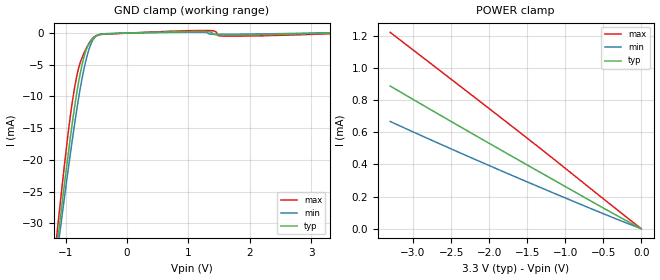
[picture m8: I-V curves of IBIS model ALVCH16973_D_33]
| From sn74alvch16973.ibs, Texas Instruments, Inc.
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[Model]   ALVCH16973_D_33
Model_type  Input
Vinl=0.8
Vinh=2.0
| variable   typ   min   max
C_comp   2.29pF   1.80pF   2.85pF
[Temperature Range]   40   100   -40
| Ambient temperature   25   85   -40
[Voltage range]   3.3   3   3.6
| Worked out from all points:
|   GND clamp passes 1 mA (typ) near -0.57 V on its own axis
[GND Clamp]
| ALVCH16973_D_33
|   Voltage   I(typ)   I(min)   I(max)
-3.3V     -230.3mA   -215.8mA   -247.5mA
-1.175V   -36.28mA   -37.42mA   -34.5mA
-1.125V   -32.14mA   -33.61mA   -29.93mA
-1.1V     -30.1mA    -31.73mA   -27.67mA
-940mV    -17.53mA   -20.04mA   -14.12mA
-815mV    -9.044mA   -11.69mA   -6.512mA
-675mV    -2.858mA   -4.436mA   -2.567mA
-590mV    -1.232mA   -1.707mA   -1.143mA
-500mV    -448.2uA   -438.6uA   -378.9uA
1.22V     242.4uA    134.2uA    415.3uA
1.57V     -286uA     -180.7uA   -464.8uA
3.3V      206.3pA    55.22uA    -106.7uA
[POWER Clamp]
| ALVCH16973_D_33
|   Voltage   I(typ)   I(min)   I(max)
-3.3V     888.3uA    667.3uA    1.222mA
-1.59V    421.1uA    309.6uA    597.1uA
-555mV    143.7uA    104.1uA    207.7uA
-48.03fV  206.3pA    943.6pA    68.36pA
